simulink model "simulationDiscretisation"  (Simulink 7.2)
settings: Solver=ode23  StartTime=0.0  StopTime=1  RelTol=1e-3
undefined symbols (not defined in the file or in its folder): h

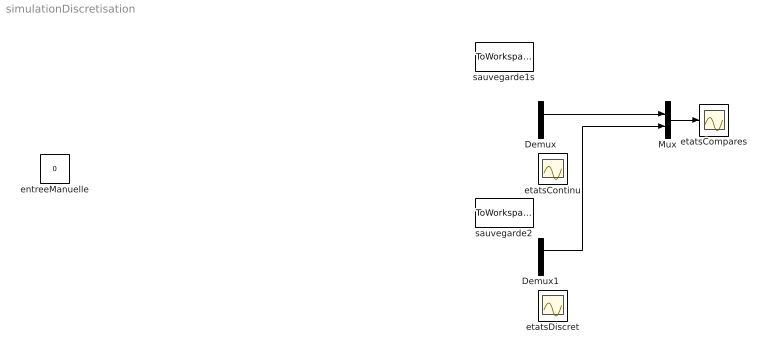
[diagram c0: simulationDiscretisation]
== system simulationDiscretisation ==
  Demux : Demux  Outputs=2
  Demux1 : Demux  Outputs=2
  Mux : Mux  Inputs=2
  entreeManuelle : Constant  Value=0  OutDataType=sfix(16)  OutScaling=2^0  SampleTime=h
  etatsCompares : Scope
  etatsContinu : Scope
  etatsDiscret : Scope
  sauvegarde1s : ToWorkspace  VariableName=etatsLin  SampleTime=-1  SaveFormat=Structure With Time
  sauvegarde2 : ToWorkspace  VariableName=etatsDisc  SampleTime=-1  SaveFormat=Structure With Time
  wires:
  Demux/1 -> Mux/1
  Demux1/1 -> Mux/2
  Mux/1 -> etatsCompares/1
